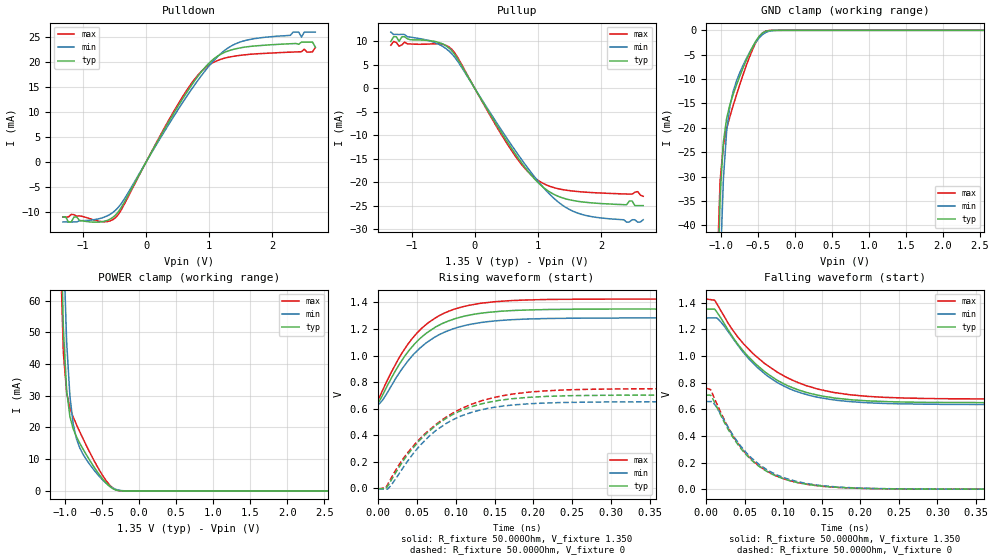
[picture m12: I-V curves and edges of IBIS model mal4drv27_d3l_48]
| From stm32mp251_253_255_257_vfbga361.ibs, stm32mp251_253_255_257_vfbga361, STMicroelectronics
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[Model] mal4drv27_d3l_48
Model_type   I/O
Polarity   Non-Inverting
Enable   Active-High
C_comp   1.684pF   1.663pF   1.711pF
C_comp_pullup   812.531fF   800.254fF   826.800fF
C_comp_pulldown   769.496fF   756.297fF   787.425fF
Vinh = 805.000mV
Vinl = 545.000mV
Vmeas = 675.000mV
Vref = 675.000mV
Rref = 50Ohms
Cref = 0pF
[Model Spec]
Vinh   805.000mV   772.000mV   855.000mV
Vinl   545.000mV   512.000mV   595.000mV
Vmeas   675.000mV   642.000mV   725.000mV
Vref   675.000mV   642.000mV   725.000mV
D_overshoot_ampl_h 0.4 NA   NA
D_overshoot_ampl_l 0.4 NA   NA
D_overshoot_area_l 110.000m NA   NA
D_overshoot_area_h 110.000m NA   NA
[Temperature Range]   25.000   125.000   -40.000
[Voltage Range]   1.350V   1.283V   1.425V
[GND Clamp Reference]   0.00V   0.00V   0.00V
[C Comp Corner]
| variable   typ   min   max
C_comp   1.684pF   1.663pF   1.711pF
C_comp_pullup   812.531fF   800.254fF   826.800fF
C_comp_pulldown   769.496fF   756.297fF   787.425fF
[Pulldown Reference]   0.00V   0.00V   0.00V
[POWER Clamp Reference]   1.350V   1.283V   1.425V
[Pullup Reference]   1.350V   1.283V   1.425V
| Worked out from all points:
|   slope of the pulldown table from 0 to 0.203 V, typ, clamps not added: 44 ohm
|   slope of the pullup table from 0 to 0.203 V, typ, clamps not added: 44.1 ohm
|   GND clamp passes 1 mA (typ) near -0.47 V on its own axis
|   POWER clamp passes 1 mA (typ) near -0.37 V on its own axis
|   rising waveform, R_fixture 50.000Ohm, V_fixture 1.350: 20-80 % time 59.4ps typ, 61.4ps min, 58.7ps max; typ from 0.648 V to 1.35 V
|   rising waveform, R_fixture 50.000Ohm, V_fixture 0: 20-80 % time 73.4ps typ, 68.9ps min, 83.6ps max; typ from -0.002 V to 0.703 V
|   falling waveform, R_fixture 50.000Ohm, V_fixture 1.350: 20-80 % time 74.5ps typ, 72.1ps min, 83.7ps max; typ from 1.35 V to 0.649 V
|   falling waveform, R_fixture 50.000Ohm, V_fixture 0: 20-80 % time 58.4ps typ, 60.8ps min, 57.8ps max; typ from 0.705 V to 0 V
[GND Clamp]
-1.318V   -672mA     -638mA     -661.1mA
-1.054V   -60.41mA   -84.99mA   -50.75mA
-1.011V   -34.02mA   -49.92mA   -30.84mA
-966.7mV  -22.91mA   -30.54mA   -23.58mA
-922.7mV  -18.04mA   -20.68mA   -20.16mA
-878.8mV  -15.25mA   -15.56mA   -17.69mA
-834.8mV  -13.14mA   -12.55mA   -15.44mA
-747mV    -9.486mA   -8.743mA   -11.21mA
-615.2mV  -4.709mA   -4.591mA   -5.504mA
-439.4mV  -562.2uA   -889.5uA   -546.1uA
-219.7mV  -954.1nA   -9.356uA   -215nA
2.68V     18.98nA    945nA      23.53nA
[Power Clamp]
-1.33V    889mA      842.2mA    872.8mA
-1.067V   94.44mA    130.9mA    77.96mA
-1.023V   51.04mA    78.45mA    43.53mA
-978.8mV  31.54mA    46.94mA    31.01mA
-934.8mV  23.45mA    29.85mA    26.15mA
-890.9mV  19.58mA    21.13mA    23.3mA
-847mV    17.11mA    16.47mA    20.93mA
-671.2mV  9.815mA    8.474mA    12.37mA
-495.5mV  3.823mA    3.529mA    4.955mA
-363.6mV  819.5uA    1.024mA    1.072mA
-187.9mV  4.227uA    28.6uA     2.566uA
2.668V    -29.12nA   -796.8nA   -15.73nA
[Pulldown]
-1.318V   -11mA      -12mA      -11mA
-1.23V    -12mA      -12mA      -11mA
-1.099V   -11mA      -12mA      -10.84mA
-747mV    -12.02mA   -11.35mA   -11.84mA
-483.3mV  -10.61mA   -9.637mA   -11.11mA
615.2mV   13.36mA    12.59mA    13.81mA
878.8mV   18.11mA    17.34mA    18.19mA
1.142V    21.27mA    21.22mA    20.37mA
1.582V    23.03mA    24.35mA    21.48mA
2.461V    24mA       25mA       22.07mA
2.636V    24mA       26mA       22.05mA
2.68V     23mA       26mA       22.93mA
[Pullup]
-1.33V    10mA       12mA       9.193mA
-1.286V   11mA       11.48mA    10mA
-1.199V   10mA       11.48mA    9mA
-1.155V   11mA       11.53mA    9.264mA
-671.2mV  10.11mA    9.945mA    9.494mA
-363.6mV  8.013mA    7.366mA    8.322mA
647mV     -14.05mA   -13.36mA   -14.53mA
910.6mV   -18.76mA   -18.23mA   -18.64mA
1.174V    -21.97mA   -22.4mA    -20.8mA
1.702V    -24.2mA    -26.89mA   -22.07mA
2.58V     -25mA      -28.52mA   -22mA
2.668V    -25mA      -28mA      -23mA
[Ramp]
R_load=50.000Ohm
dV/dt_r   421.200mV/67.500ps  389.998mV/65.500ps  450.000mV/72.500ps
dV/dt_f   421.200mV/67.500ps  389.999mV/67.500ps  450.000mV/72.000ps
[Rising waveform]
R_fixture=50.000Ohm
V_fixture=1.350
V_fixture_min=1.283
V_fixture_max=1.425
0s        648mV      632mV      671mV
8ps       729mV      684mV      768mV
28ps      941mV      877mV      993mV
37ps      1.018V     949mV      1.075V
50ps      1.106V     1.035V     1.17V
74ps      1.215V     1.142V     1.285V
108ps     1.292V     1.22V      1.366V
144ps     1.326V     1.257V     1.401V
196ps     1.344V     1.276V     1.419V
500ps     1.35V      1.283V     1.425V
[Rising waveform]
R_fixture=50.000Ohm
V_fixture=0
0s        -1.689mV   -5.298mV   -3.722mV
10ps      -1.689mV   -5.298mV   6.556mV
14ps      34.19mV    6.39mV     49.15mV
39ps      262mV      215mV      277mV
56ps      378mV      337mV      387mV
75ps      478mV      439mV      484mV
109ps     591mV      550mV      606mV
151ps     658mV      612mV      687mV
242ps     697mV      647mV      742mV
510ps     703mV      652mV      751mV
[Falling waveform]
R_fixture=50.000Ohm
V_fixture=1.350
V_fixture_min=1.283
V_fixture_max=1.425
0s        1.351V     1.284V     1.426V
11ps      1.351V     1.284V     1.418V
15ps      1.32V      1.279V     1.38V
41ps      1.088V     1.08V      1.142V
79ps      867mV      851mV      929mV
109ps     768mV      751mV      826mV
146ps     704mV      688mV      749mV
188ps     671mV      656mV      707mV
257ps     654mV      639mV      683mV
511ps     649mV      635mV      676mV
[Falling waveform]
R_fixture=50.000Ohm
V_fixture=0
0s        705mV      657mV      758mV
6ps       705mV      657mV      746mV
11ps      650mV      637mV      679mV
32ps      415mV      431mV      428mV
54ps      245mV      262mV      251mV
79ps      132mV      145mV      134mV
115ps     53.77mV    61.35mV    53.72mV
157ps     18.75mV    22.25mV    18.56mV
206ps     5.49mV     6.747mV    5.188mV
506ps     486.3nV    7.07uV     289nV
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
